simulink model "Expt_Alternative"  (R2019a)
settings: Solver=VariableStepAuto  StartTime=0  StopTime=100  RelTol=1e-3

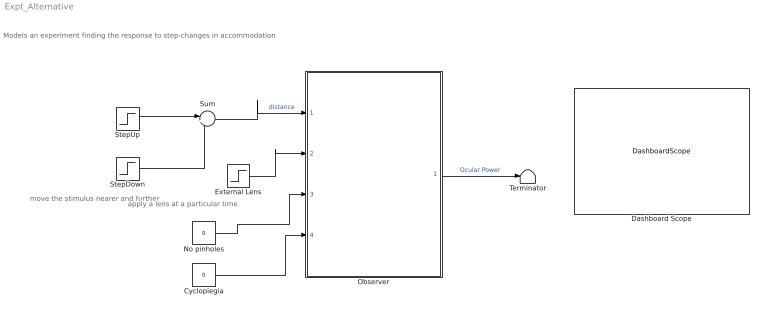
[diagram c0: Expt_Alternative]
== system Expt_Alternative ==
  note: Models an experiment finding the response to step-changes in accommodation
  note: move the stimulus nearer and further
  note: apply a lens at a particular time
  Cycloplegia : Constant  Value=0
  Dashboard Scope : DashboardScope
  External Lens : Step  Time=0  After=0  SampleTime=0
  No pinholes : Constant  Value=0
  Observer : ModelReference  ModelNameDialog=SimplifiedAccommodationModel_Alternative.slx  SimulationMode=Normal  ModelReferenceVersion=1.36
  StepDown : Step  Time=20  After=-2  SampleTime=0
  StepUp : Step  Time=10  Before=3  After=4  SampleTime=0
  Sum : Sum  Inputs=|++
  Terminator : Terminator
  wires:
  No pinholes/1 -> Observer/3
  StepUp/1 -> Sum/1
  Observer/1 -> Terminator/1  "Ocular Power"
  Sum/1 -> Observer/1  "distance"
  StepDown/1 -> Sum/2
  External Lens/1 -> Observer/2
  Cycloplegia/1 -> Observer/4
